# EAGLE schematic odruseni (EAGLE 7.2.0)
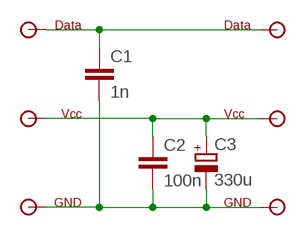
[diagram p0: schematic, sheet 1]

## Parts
C1  1n  C-EUC1206  [C1206]
C2  100n  C-EUC1206  [C1206]
C3  330u  CPOL-EUSMCD  [SMC_D]
U$1  Data  CON_1  [CON_1]
U$2  Vcc  CON_1  [CON_1]
U$3  GND  CON_1  [CON_1]
U$4  GND  CON_1  [CON_1]
U$5  Vcc  CON_1  [CON_1]
U$6  Data  CON_1  [CON_1]

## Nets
N$2: C1.2 C2.2 C3.- U$3.P$1 U$4.P$1
N$3: C2.1 C3.+ U$2.P$1 U$5.P$1
N$4: C1.1 U$1.P$1 U$6.P$1

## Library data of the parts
C1 C2 = rcl:C-EU: CAPACITOR, European symbol
C3 = rcl:CPOL-EU: POLARIZED CAPACITOR, European symbol
U$1-U$6 = arduino:CON_1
